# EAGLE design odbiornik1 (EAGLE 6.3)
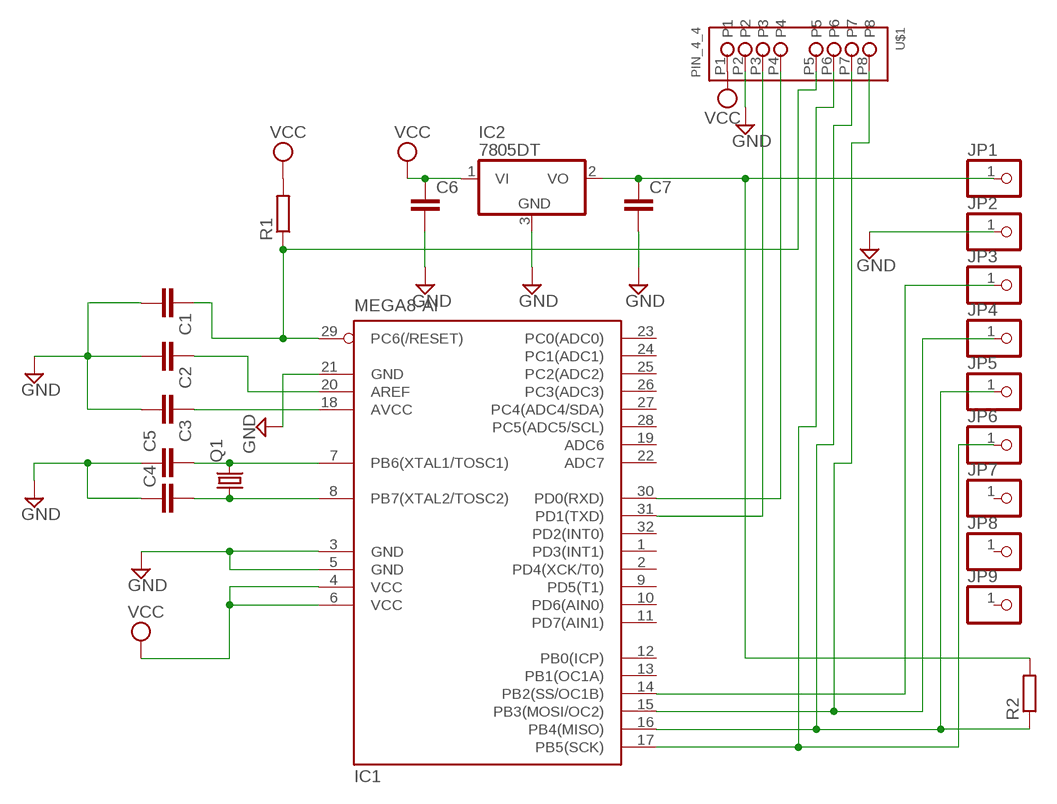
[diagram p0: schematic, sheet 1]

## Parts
C1  C-EUC0805  [C0805]
C2  C-EUC0805  [C0805]
C3  C-EUC0805  [C0805]
C4  C-EUC0805  [C0805]
C5  C-EUC0805  [C0805]
C6  C-EUC0805  [C0805]
C7  C-EUC0805  [C0805]
IC1  MEGA8-AI  [TQFP32-08]
IC2  7805DT  [TO252]
JP1  PINHD-1X1  [1X01]
JP2  PINHD-1X1  [1X01]
JP3  PINHD-1X1  [1X01]
JP4  PINHD-1X1  [1X01]
JP5  PINHD-1X1  [1X01]
JP6  PINHD-1X1  [1X01]
JP7  PINHD-1X1  [1X01]
JP8  PINHD-1X1  [1X01]
JP9  PINHD-1X1  [1X01]
Q1  CRYSTALHC49UP  [HC49UP]
R1  R-EU_M0805  [M0805]
R2  R-EU_R0805  [R0805]
U$1  PIN_4_4  [PIN_4_4]

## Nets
GND: C1.2 C2.2 C3.2 C4.1 C5.1 C6.2 C7.2 IC1.3(GND) IC1.5(GND) IC1.21(GND) IC2.3(GND) JP2.1 U$1.P2
N$1: C3.1 IC1.18(AVCC)
N$2: C2.1 IC1.20(AREF)
N$3: C1.1 IC1.29(PC6(/RESET)) R1.1 U$1.P5
N$4: C5.2 IC1.7(PB6(XTAL1/TOSC1)) Q1.2
N$5: C4.2 IC1.8(PB7(XTAL2/TOSC2)) Q1.1
N$6: IC1.17(PB5(SCK)) JP6.1 U$1.P6
N$7: IC1.16(PB4(MISO)) JP5.1 R2.1 U$1.P7
N$8: IC1.15(PB3(MOSI/OC2)) JP4.1 U$1.P8
N$9: IC1.14(PB2(SS/OC1B)) JP3.1
N$10: C7.1 IC2.2(VO) JP1.1 R2.2
N$11: IC1.31(PD1(TXD)) U$1.P3
N$12: IC1.30(PD0(RXD)) U$1.P4
VCC: C6.1 IC1.4(VCC) IC1.6(VCC) IC2.1(VI) R1.2 U$1.P1
Unconnected: IC1.1(PD3(INT1)) IC1.2(PD4(XCK/T0)) IC1.9(PD5(T1)) IC1.10(PD6(AIN0)) IC1.11(PD7(AIN1)) IC1.12(PB0(ICP)) IC1.13(PB1(OC1A)) IC1.19(ADC6) IC1.22(ADC7) IC1.23(PC0(ADC0)) IC1.24(PC1(ADC1)) IC1.25(PC2(ADC2)) IC1.26(PC3(ADC3)) IC1.27(PC4(ADC4/SDA)) IC1.28(PC5(ADC5/SCL)) IC1.32(PD2(INT0)) JP7.1 JP8.1 JP9.1

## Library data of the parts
C1-C7 = rcl:C-EU: CAPACITOR, European symbol
IC1 = atmel:MEGA8: MICROCONTROLLER 8 Kbytes FLASH, 1 kbytes SRAM, 512 bytes EEPROM, USART, 6-channel 10 bit ADC, 2-channel 8 bit ADC Pin compatible with Atmega48, ATMega88, ATMega168 Source: avr.lbr
IC2 = linear:78*: Positive VOLTAGE REGULATOR Source: http://cache.national.com/ds/LM/LM78L05.pdf http://www.fairchildsemi.com/ds/LM/LM7805.pdf
JP1-JP9 = pinhead:PINHD-1X1: PIN HEADER
Q1 = crystal:CRYSTAL: CRYSTAL
R1 R2 = rcl:R-EU_: RESISTOR, European symbol
U$1 = pin_4_4:PIN_4_4

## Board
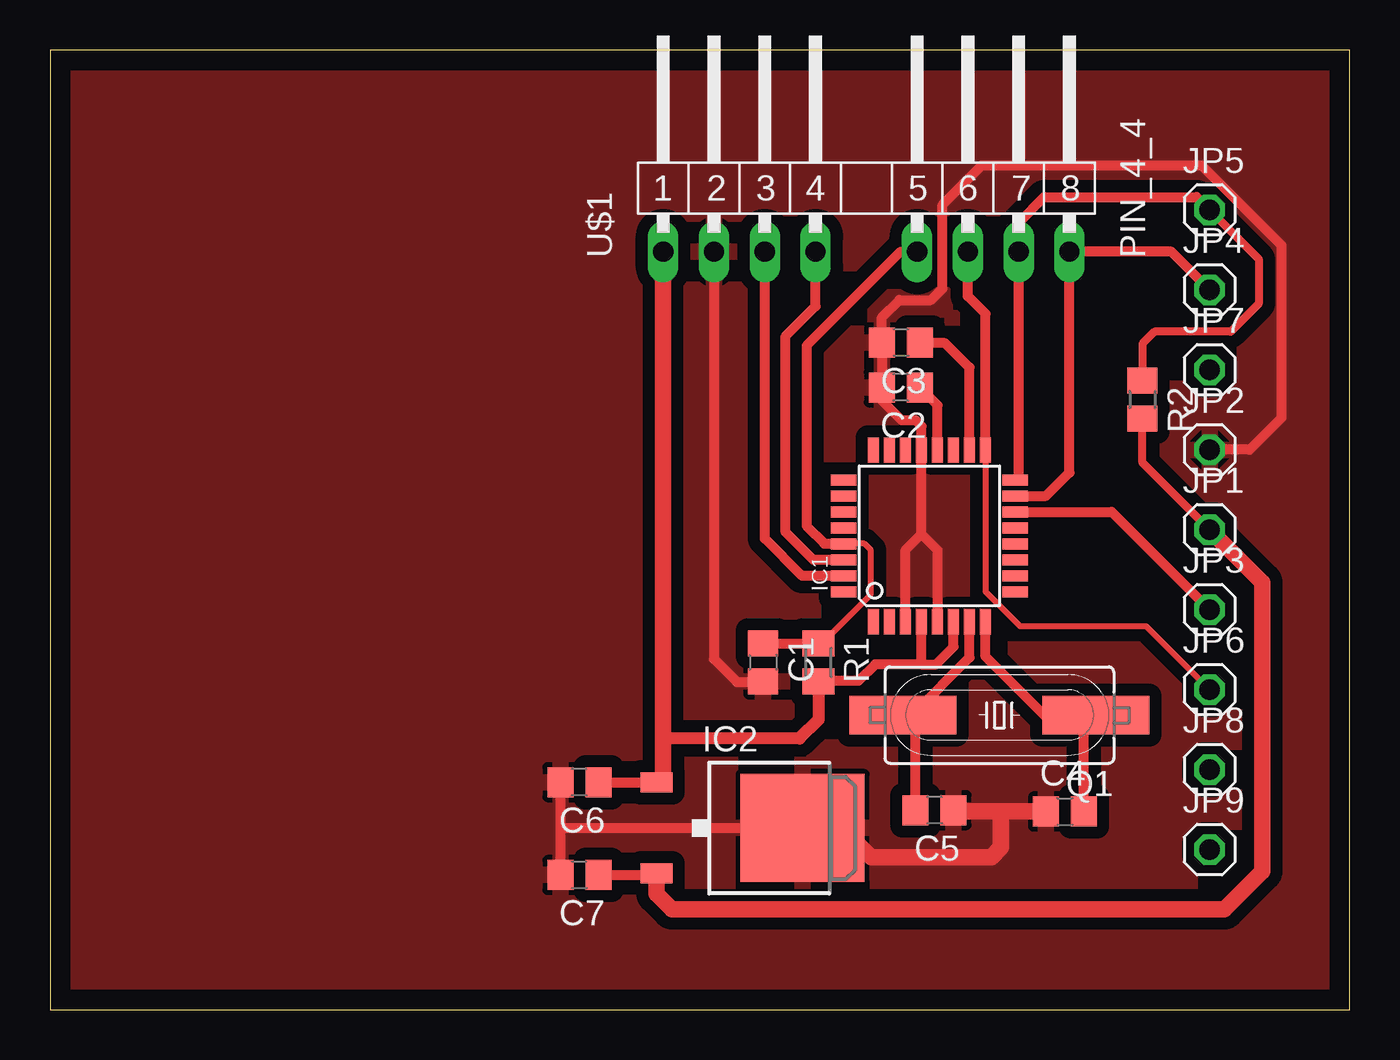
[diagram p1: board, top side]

Size 65 x 48 mm. Coordinates in mm from the lower left corner, seen from the top.
Outline: 0,0 65,0 65,48 0,48 0,0
Copper layers (1*16): Top 0.035mm / dielectric 1.5mm / Bottom 0.035mm
Design rules "default": minimum track width 10mil, minimum drill 24mil, track to track 8mil, track to pad 8mil, pad to pad 8mil, via to via 8mil, smd to smd 8mil, copper to edge 40mil, drill to drill 8mil, minimum pad ring 10mil, minimum via ring 8mil, stop-mask expansion 4mil, vias tented up to drill 0mil, thermal gap 10mil

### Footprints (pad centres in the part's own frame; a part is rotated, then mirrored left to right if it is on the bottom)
C0805 = smd 1.3 x 1.5: 1 -0.95,0; 2 0.95,0
TQFP32-08 = smd 1.27 x 0.559: 1 -4.293,2.8; 2 -4.293,2; 3 -4.293,1.2; 4 -4.293,0.4; 5 -4.293,-0.4; 6 -4.293,-1.2; 7 -4.293,-2; 8 -4.293,-2.8; 17 4.293,-2.8; 18 4.293,-2; 19 4.293,-1.2; 20 4.293,-0.4; 21 4.293,0.4; 22 4.293,1.2; 23 4.293,2; 24 4.293,2.8 | smd 0.559 x 1.27: 9 -2.8,-4.293; 10 -2,-4.293; 11 -1.2,-4.293; 12 -0.4,-4.293; 13 0.4,-4.293; 14 1.2,-4.293; 15 2,-4.293; 16 2.8,-4.293; 25 2.8,4.293; 26 2,4.293; 27 1.2,4.293; 28 0.4,4.293; 29 -0.4,4.293; 30 -1.2,4.293; 31 -2,4.293; 32 -2.8,4.293
TO252 = smd 1 x 1.6: 1 -2.28,-4.8; 2 2.28,-4.8 | smd 5.4 x 6.2: 3 0,2.5
1X01 = drill 1.016 octagon: 1 0,0
HC49UP = smd 5.334 x 1.93: 1 -4.826,0; 2 4.826,0
M0805 = smd 1.3 x 1.6: 1 -0.95,0; 2 0.95,0
R0805 = smd 1.3 x 1.5: 1 -0.95,0; 2 0.95,0
PIN_4_4 = drill 1.016 long: P1 -10.16,0.318; P2 -7.62,0.318; P3 -5.08,0.318; P4 -2.54,0.318; P5 2.54,0.318; P6 5.08,0.318; P7 7.62,0.318; P8 10.16,0.318

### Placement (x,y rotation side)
C1  35.67,17.37 270 top
C2  42.55,31.12 180 top
C3  42.57,33.35 180 top
C4  50.77,9.91 0 top
C5  44.25,9.97 180 top
C6  26.48,11.37 180 top
C7  26.48,6.73 180 top
IC1  43.99,23.69 90 top
IC2  35.15,9.08 270 top
JP1  58,24 0 top
JP2  58,28 0 top
JP3  58,20 0 top
JP4  58,36 0 top
JP5  58,40 0 top
JP6  58,16 0 top
JP7  58,32 0 top
JP8  58,12 0 top
JP9  58,8 0 top
Q1  47.49,14.73 180 top
R1  38.44,17.37 270 top
R2  54.64,30.51 270 top
U$1  40.83,37.59 0 top

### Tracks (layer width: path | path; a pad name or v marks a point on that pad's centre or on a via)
GND
  Top 0.508: IC1.3 42.79,22.98 43.59,23.78 | 43.59,23.78 IC1.21 43.59,29.18 43.31,29.46 42.61,29.46 41.53,30.54 41.53,31.05 C2.2 41.62,31.14 C3.2 41.62,34.64 42.48,35.5 44.07,35.5 44.64,36.07 44.64,40.26 46.61,42.23 57.59,42.23 61.59,38.23 61.59,29.59 60.01,28 JP2.1 | IC1.5 44.39,22.98 43.59,23.78 | C7.2 25.53,9.02 | 25.53,9.02 C6.2 | 25.53,9.02 25.59,9.08 IC2.3 | C1.2 35.63,16.38 34.35,16.38 33.21,17.53 U$1.P2
  Top 0.61: 58,28.03 JP2.1
  Top 0.813: C4.1 47.56,9.91 | 47.56,9.91 45.7,9.91 C5.1 | IC2.3 39.62,9.08 41.08,7.62 47.08,7.62 47.56,8.1 47.56,9.91
  pour Top (isolate 0.61): -0.32,48.32 -0.32,-0.38 65.47,-0.38 65.47,48.7 -0.32,48.7
N$1
  Top 0.508: IC1.18 45.99,32.12 44.77,33.34 43.99,33.34 C3.1
N$2
  Top 0.508: IC1.20 44.39,30.23 C2.1
N$3
  Top 0.305: 38.61,18.32 41.05,20.77 41.05,22.99 40.73,23.3 39.71,23.3
  Top 0.406: R1.1 38.61,18.32 | 39.71,23.3 IC1.29
  Top 0.508: C1.1 R1.1 | IC1.29 39.69,23.3 38.73,23.3 37.85,24.19 37.85,33.21 42.55,37.91 U$1.P5
N$4
  Top 0.508: 43.18,14.8 42.73,14.8 Q1.2 | 42.85,14.46 43.18,14.8 | IC1.7 45.99,17.61 43.18,14.8 | C5.2 43.3,14.68 43.18,14.8
N$5
  Top 0.508: 52.17,14.58 Q1.1 52.19,14.61 51.31,14.61 | IC1.8 46.79,17.66 49.85,14.61 51.31,14.61 | C4.2 51.72,14.2 51.31,14.61
N$6
  Top 0.305: IC1.17 46.79,20.9 48.51,19.18 54.82,19.18 JP6.1
  Top 0.508: 57.98,16 JP6.1 | IC1.17 46.79,34.81 45.91,35.69 U$1.P6
N$7
  Top 0.406: R2.1 54.64,33.3 55.24,33.91 59.05,33.91 60.45,35.31 60.45,37.55 JP5.1
  Top 0.508: JP5.1 57.36,40.64 49.72,40.64 48.45,39.37 U$1.P7 48.45,26.66 IC1.16
N$8
  Top 0.508: IC1.15 49.82,25.69 50.99,26.86 U$1.P8 56.09,37.91 JP4.1
N$9
  Top 0.508: JP3.1 53.11,24.89 IC1.14
N$10
  Top 0.406: R2.2 54.64,27.36 JP1.1
  Top 0.508: C7.1 30.27,6.73 IC2.2
  Top 0.813: IC2.2 30.35,5.79 31.11,5.02 58.74,5.02 60.64,6.92 60.64,21.36 JP1.1
N$11
  Top 0.508: IC1.31 37.62,21.69 35.75,23.56 U$1.P3
N$12
  Top 0.508: IC1.30 38.18,22.49 36.8,23.88 36.8,33.69 38.29,35.18 U$1.P4
VCC
  Top 0.508: IC1.6 45.19,18.14 44.32,17.27 43.56,17.27 | IC1.4 43.59,17.3 43.56,17.27 | C6.1 IC2.1 | 43.56,17.27 41.27,17.27 40.45,16.45 38.46,16.45 R1.2
  Top 0.61: R1.2 38.44,14.5 37.5,13.56 30.73,13.56 30.67,13.62
  Top 0.813: IC2.1 30.67,11.69 30.67,13.62 U$1.P1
